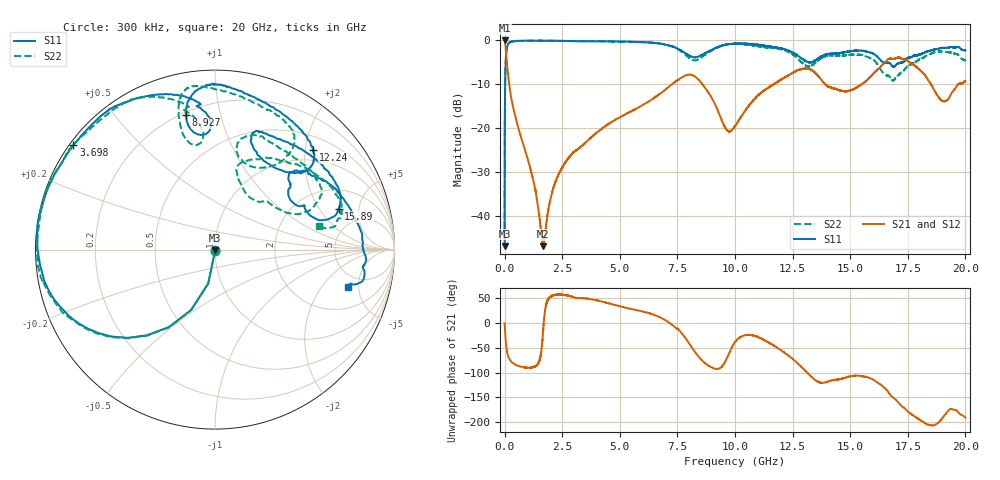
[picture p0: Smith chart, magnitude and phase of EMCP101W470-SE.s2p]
!EMCP101W470
!Johanson Technology Inc.
!www.johansontechnology.com
!Test Board Conditions:
!Substrate Type  RO4350B
!Substrate Thickness  10 mil
!Substrate Dk  3.66
!TL Type: GCPW
!TL Trace Width  20 mil
!TL Gap  10 mil
!PART MODE SINGLE ENDED (AKA BYPASS)
!DUT TOPOLOGY	SERIES-SHUNT
# MHz S  dB  R 50
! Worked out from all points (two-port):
!   20001 points, 300 kHz to 20 GHz, reference 50 ohm
!   highest |S21| = 0.01 dB at 300 kHz (marker M1); lowest = -47.0 dB at 1.671 GHz (marker M2)
!   |S21| within 3 dB of the highest: start of sweep to 66.78 MHz
!   lowest |S11| = -46.9 dB at 300 kHz (marker M3), VSWR 1.01, Z = 50 - j0.448 ohm
!   |S11| at or under -10 dB: start of sweep to 22.62 MHz
!   |S22| runs from -45.4 to 0.0 dB; largest |S21 - S12| = 0.013
!   S11 on the Smith chart (normalised r, x): 300 kHz: 1.00, -0.01; 3.698 GHz: 0.01, +0.33; 8.927 GHz: 0.22, +0.78; 12.24 GHz: 0.76, +2.16; 15.89 GHz: 3.19, +3.05; 20 GHz: 3.62, -3.72
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0.3  -46.95 -84.8  0.01 -0.3  -0.01 -0.2  -45.41 -83.1
102.298  -1.64 -147.6  -5.23 -57.0  -5.25 -57.0  -1.58 -147.4
160.298  -0.81 -158.6  -8.30 -67.8  -8.36 -67.8  -0.69 -158.5
562.292  -0.13 -179.3  -19.36 -85.8  -19.36 -85.9  -0.07 -176.3
1252.281  -0.03 170.8  -32.04 -88.4  -32.02 -88.2  -0.08 172.0
1671.275  -0.05 166.1  -46.97 -15.7  -46.81 -15.9  -0.04 165.6
2265.266  -0.06 160.1  -31.50 57.5  -31.47 57.6  -0.08 157.9
3334.25  -0.16 148.8  -24.13 50.6  -24.10 50.7  -0.15 148.8
3698.245  -0.18 143.6  -22.40 49.0  -22.39 49.1  -0.13 146.9
6667.2  -0.66 111.7  -12.45 13.6  -12.46 13.3  -0.64 113.4
8022.18  -3.46 92.3  -7.80 -41.8  -7.84 -41.6  -4.01 96.0
8927.166  -2.31 102.3  -12.55 -88.0  -12.51 -88.0  -2.45 105.3
10000.15  -0.74 91.8  -19.56 -38.4  -19.51 -38.2  -0.74 97.8
12243.12  -2.17 45.5  -8.18 -63.2  -8.25 -62.6  -2.39 54.1
13334.1  -4.97 61.2  -6.80 -109.2  -6.75 -108.8  -5.69 73.1
14283.09  -3.07 64.7  -10.96 -115.1  -10.84 -115.0  -3.44 63.3
15892.06  -2.80 18.2  -8.21 -111.9  -8.21 -112.2  -4.06 24.9
16667.05  -5.10 26.2  -4.20 -140.2  -4.23 -139.2  -8.09 43.2
17349.04  -4.66 45.1  -4.33 -171.8  -4.34 -171.4  -6.73 75.2
18110.03  -3.02 33.9  -7.16 162.1  -7.09 161.7  -4.09 52.1
19049.01  -1.70 3.7  -13.88 171.1  -13.86 171.2  -2.58 18.7
20000  -2.31 -16.0  -9.29 168.8  -9.27 168.2  -4.59 12.9
